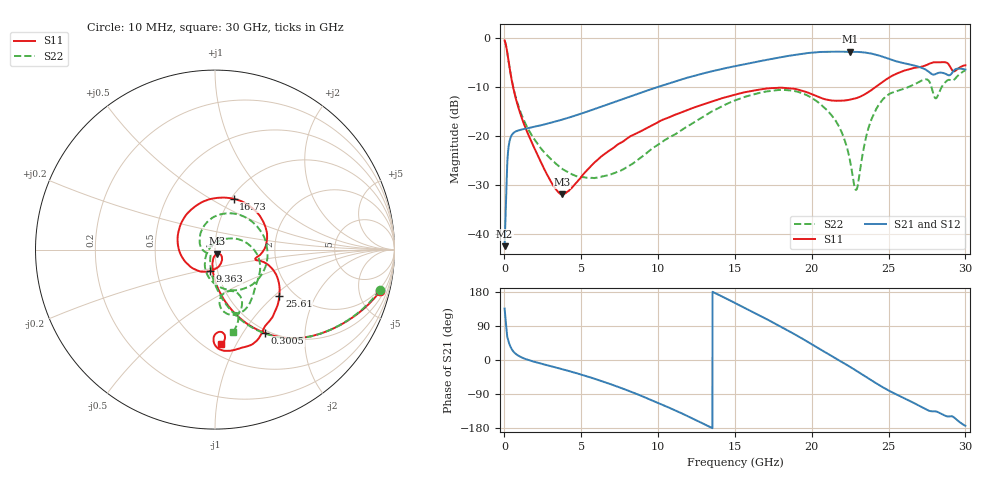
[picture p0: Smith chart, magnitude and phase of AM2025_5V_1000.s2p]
!Keysight Technologies,N5245B,MY58422270,A.16.20.02
!Date: Tuesday, July 14, 2026 01:06:28
!Correction: S11(C  2-Port  )
!S21(C  2-Port  )
!S12(C  2-Port  )
!S22(C  2-Port  )
!S2P File: Measurements: S11, S21, S12, S22:
# Hz S  dB  R 50
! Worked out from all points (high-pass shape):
!   3201 points, 10 MHz to 30 GHz, reference 50 ohm
!   highest |S21| = -2.76 dB at 22.5 GHz (marker M1); lowest = -42.4 dB at 10 MHz (marker M2)
!   |S21| within 3 dB of the highest: 14.91 GHz to 26.89 GHz (11.98 GHz wide, 57.3 % of centre)
!   lowest |S11| = -31.9 dB at 3.749 GHz (marker M3), VSWR 1.05, Z = 50.9 - j2.4 ohm
!   |S11| at or under -10 dB: 565.2 MHz to 24.13 GHz (23.57 GHz wide, 191 % of centre)
!   |S22| runs from -30.9 to -0.5 dB; largest |S21 - S12| = 0.013
!   S11 on the Smith chart (normalised r, x): 10 MHz: 1.67, -7.70; 300.5 MHz: 0.96, -1.26; 9.363 GHz: 0.92, -0.22; 16.73 GHz: 1.03, +0.64; 25.61 GHz: 1.68, -1.08; 30 GHz: 0.60, -0.87
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1e7  -0.46 -14.1  -42.40 135.7  -36.36 87.1  -0.48 -13.7
3.005281e8  -5.35 -59.3  -21.48 44.4  -21.45 44.4  -5.33 -59.5
6.379156e8  -11.02 -80.0  -19.20 19.9  -19.20 20.0  -10.86 -80.7
1.472012e9  -19.08 -96.9  -18.38 1.2  -18.37 1.2  -18.09 -99.6
3.749378e9  -31.86 -67.2  -16.60 -24.2  -16.60 -24.2  -26.61 -123.1
5.014581e9  -28.20 -41.8  -15.36 -38.8  -15.34 -38.8  -28.30 -131.7
9.363131e9  -18.15 -104.1  -10.60 -102.2  -10.59 -102.3  -23.14 -179.2
1.000979e10  -17.10 -117.8  -9.92 -113.2  -9.93 -113.3  -21.69 167.5
1.228716e10  -14.19 -173.7  -7.72 -155.2  -7.71 -155.3  -17.27 120.2
1.5005e10  -11.53 114.2  -5.70 150.5  -5.70 150.5  -12.68 58.2
1.672942e10  -10.41 69.8  -4.62 115.0  -4.61 114.9  -11.05 16.8
1.848197e10  -10.19 27.4  -3.61 77.0  -3.61 76.9  -10.62 -27.6
2.000958e10  -11.42 -1.8  -2.93 41.5  -2.92 41.4  -12.20 -67.2
2.164966e10  -12.76 -12.7  -2.76 2.1  -2.76 2.1  -17.30 -110.9
2.25025e10  -12.51 -14.4  -2.76 -18.3  -2.76 -18.3  -25.12 -150.2
2.292423e10  -12.20 -14.2  -2.79 -28.9  -2.78 -28.9  -30.79 124.7
2.379582e10  -10.76 -14.8  -3.08 -51.3  -3.08 -51.3  -17.32 26.0
2.500479e10  -8.08 -26.3  -4.19 -80.5  -4.19 -80.6  -11.47 -19.7
2.561396e10  -7.10 -35.7  -4.81 -92.8  -4.81 -92.8  -10.69 -35.4
2.745085e10  -5.50 -60.4  -6.47 -130.6  -6.46 -130.6  -8.39 -70.7
2.809751e10  -4.92 -72.2  -7.27 -135.8  -7.27 -135.8  -12.24 -71.5
3e10  -5.53 -86.2  -6.39 -173.5  -6.35 -173.5  -6.56 -77.7
